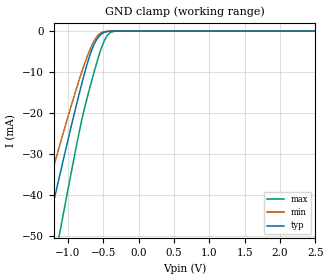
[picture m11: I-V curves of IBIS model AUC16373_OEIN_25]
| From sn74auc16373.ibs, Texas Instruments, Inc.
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[Model]   AUC16373_OEIN_25
Model_type  Input
Vinl=0.7
Vinh=1.7
| variable   typ   min   max
C_comp   2.45pF   1.96pF   2.83pF
[Temperature Range]   40   100   -40
| Ambient temperature   25   85   -40
[Voltage range]   2.5   2.3   2.7
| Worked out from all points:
|   GND clamp passes 1 mA (typ) near -0.55 V on its own axis
[GND Clamp]
| AUC16373_OEIN_25
|   Voltage   I(typ)   I(min)   I(max)
-3.6V     -226.6mA   -190.3mA   -271.8mA
-1.455V   -60.71mA   -48.79mA   -79.87mA
-1.295V   -48.52mA   -38.74mA   -65.35mA
-1.105V   -34.25mA   -27.09mA   -48.1mA
-850mV    -15.85mA   -12.35mA   -25.34mA
-785mV    -11.51mA   -8.949mA   -20.15mA
-725mV    -7.81mA    -6.074mA   -16.01mA
-625mV    -3.071mA   -2.25mA    -9.633mA
-520mV    -618.6uA   -332uA     -3.783mA
-430mV    -73.2uA    -35.47uA   -776.9uA
-325mV    -3.339uA   -2.035uA   -30.74uA
2.5V      313.9pA    402pA      470.4pA
